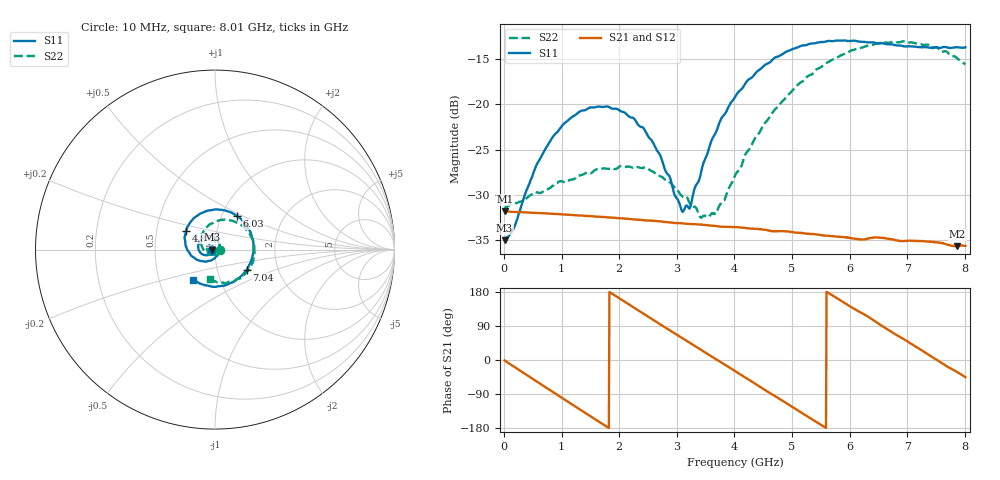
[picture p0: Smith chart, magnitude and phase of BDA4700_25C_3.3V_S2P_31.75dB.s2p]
!Agilent Technologies,E5071B,MY42404982,A.09.10
!Date: Mon Oct 20 18:16:26 2025
!Data & Calibration Information:
!Freq	S11:SOLT2(ON)	S21:SOLT2(ON)	S12:SOLT2(ON)	S22:SOLT2(ON)
# Hz S RI R 50
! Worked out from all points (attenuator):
!   801 points, 10 MHz to 8.01 GHz, reference 50 ohm
!   highest |S21| = -31.78 dB at 20 MHz (marker M1); lowest = -35.6 dB at 7.87 GHz (marker M2)
!   lowest |S11| = -35.0 dB at 10 MHz (marker M3), VSWR 1.04, Z = 48.3 - j0.0891 ohm
!   |S11| at or under -10 dB: start of sweep to end of sweep
!   |S22| runs from -32.5 to -13.0 dB; largest |S21 - S12| = 0.00033
!   S11 on the Smith chart (normalised r, x): 10 MHz: 0.97, -0.00; 4.87 GHz: 0.71, +0.16; 6.03 GHz: 1.18, +0.47; 7.04 GHz: 1.39, -0.32; 8.01 GHz: 0.74, -0.26
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1e7  -0.0177 -0.000923  0.0257 -0.000511  0.0257 -0.000544  0.0272 -0.00077
2e7  -0.0181 -0.00146  0.0257 -0.000937  0.0257 -0.00101  0.0271 -0.00105
1.6e8  -0.0183 -0.00907  0.0245 -0.00719  0.0245 -0.00715  0.0273 -0.00773
5.5e8  -0.035 -0.0287  0.0144 -0.0206  0.0145 -0.0207  0.0159 -0.0287
7.7e8  -0.0516 -0.0316  0.00577 -0.0243  0.00575 -0.0243  0.00124 -0.0342
1.35e9  -0.0923 0.00156  -0.0168 -0.0177  -0.0168 -0.0176  -0.0364 -0.0183
2.09e9  -0.056 0.0708  -0.0211 0.0102  -0.0211 0.0102  -0.0297 0.034
2.68e9  0.0124 0.0529  -0.00288 0.0224  -0.00295 0.0224  0.0126 0.0384
3.08e9  0.0261 0.00233  0.0114 0.019  0.0112 0.019  0.0281 0.0139
3.21e9  0.0222 -0.0149  0.015 0.016  0.015 0.016  0.0288 0.00491
3.42e9  0.00328 -0.042  0.0194 0.00978  0.0194 0.0098  0.0207 -0.0116
3.66e9  -0.0285 -0.0621  0.0213 0.00147  0.0213 0.00144  0.00526 -0.0243
4.01e9  -0.0925 -0.0592  0.0184 -0.0103  0.0184 -0.0102  -0.0309 -0.0259
4.37e9  -0.1489 -0.0104  0.00923 -0.0184  0.00925 -0.0185  -0.0662 0.00192
4.87e9  -0.1608 0.1063  -0.00711 -0.0186  -0.00701 -0.0187  -0.074 0.0774
5.35e9  -0.0769 0.2028  -0.0177 -0.00764  -0.0177 -0.00774  -0.016 0.146
6.03e9  0.1228 0.1875  -0.0138 0.0119  -0.014 0.0119  0.137 0.1442
6.68e9  0.2145 0.00393  0.00353 0.0177  0.00362 0.0177  0.219 0.000841
7.04e9  0.1769 -0.1121  0.0124 0.0127  0.0124 0.0126  0.1976 -0.0954
7.47e9  0.0575 -0.1989  0.0174 0.00139  0.0174 0.00133  0.1084 -0.1747
7.87e9  -0.0791 -0.1909  0.014 -0.0087  0.0141 -0.00881  0.00657 -0.1795
8.01e9  -0.1221 -0.1666  0.0116 -0.0118  0.0117 -0.0117  -0.0293 -0.1636
